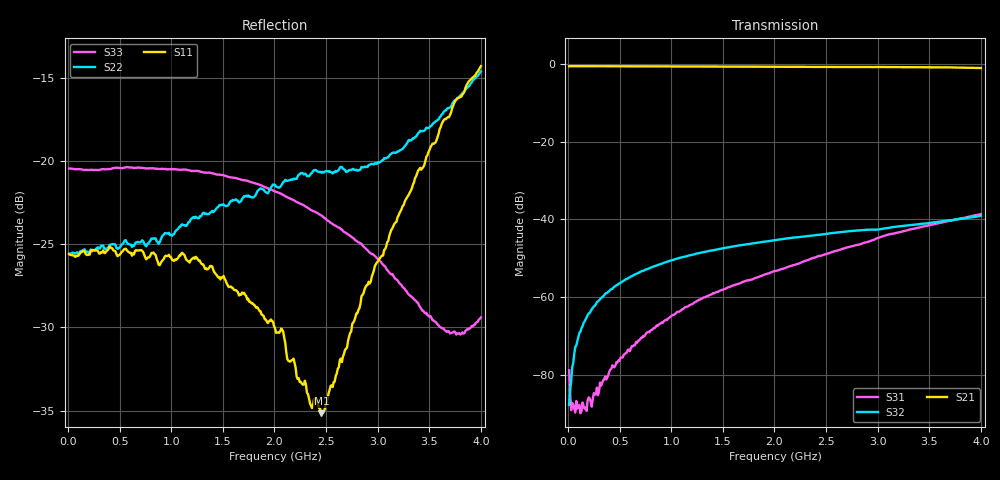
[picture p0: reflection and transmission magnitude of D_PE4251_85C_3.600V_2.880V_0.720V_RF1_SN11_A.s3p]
! Device ID: PE4251_SoldCshunt_081809
! Dir: c:\Test Bench Repositories\Bench_Software_CVI_Version_8\trunk\PSC 4Port_VNA Bench\datalog\4250\TEST\PE4251_SoldCshunt_081809\85C\3p600000\RF1
! Serial: 11
! Insertion: A
! Temp: 85C
! VDD: 3.600
! Control_Hi: 80.000
! Control_Lo: 20.000
! Logic State: RF1
! Port 1: RFC
! Port 2: RF1
! Port 3: RF2
! V1 = 0.72
! V2 = 2.88
! V3 = 0.72
! IDD: 5.518780e-05
! FILE NAME
! DATE 08/18/09  20:17
! CORRECTED  DATA
#  Hz  S  RI  R  50.00
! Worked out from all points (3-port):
!   401 points, 10 MHz to 4 GHz, reference 50 ohm
!   strongest paths, dB at 10 MHz, 1.008 GHz, 2.005 GHz, 3.002 GHz, 4 GHz:
!     S21: -0.6, -0.7, -0.8, -0.8, -1.1
!     S32: -87.7, -50.5, -45.4, -42.6, -39.1
!     S31: -78.8, -64.7, -53.3, -44.8, -38.6
!   lowest |S11| = -35.2 dB at 2.454 GHz (marker M1), VSWR 1.04, Z = 49.9 - j1.74 ohm
!   |S11| at or under -10 dB: start of sweep to end of sweep
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1e7  0.0526 0.000196  0.9309 -0.0035  8e-05 -2.85e-05
     0.9305 -0.00483  0.0525 0.000111  8.77e-05 -4.46e-05
     0.00011 3.15e-05  3.14e-05 -2.66e-05  0.0951 -0.000197
8.98e7  0.0521 -0.00168  0.9321 -0.0316  2.79e-05 -2.07e-05
        0.9314 -0.0315  0.0532 -0.00147  5.13e-05 0.000271
        2.69e-05 -2.53e-05  3.39e-05 0.000271  0.0947 -0.00193
1.696e8  0.0527 -0.000111  0.9298 -0.0584  1.66e-05 -3.75e-05
         0.9296 -0.0578  0.0537 3.84e-05  5.3e-05 0.000517
         1.05e-05 -3.66e-05  6.16e-05 0.000513  0.0942 -0.00379
3.79075e8  0.0537 -0.00419  0.9216 -0.127  -5.72e-05 -6.99e-05
           0.9208 -0.1271  0.0542 -0.00332  0.000103 0.00113
           -5.84e-05 -7.12e-05  9.56e-05 0.00113  0.0941 -0.00983
4.78825e8  0.0515 -0.00605  0.9148 -0.1604  -0.00012 -7.59e-05
           0.9144 -0.1608  0.0542 -0.00586  0.000146 0.00144
           -0.000116 -8.71e-05  0.000139 0.00143  0.0949 -0.012
1.14715e9  0.0472 -0.0178  0.8482 -0.3678  -0.000737 -7.79e-05
           0.848 -0.3673  0.0608 -0.0197  0.000556 0.00332
           -0.000745 -7.49e-05  0.000559 0.00332  0.0911 -0.0241
2.005e9  0.0259 -0.0179  0.7026 -0.5829  -0.00215 0.000146
         0.7029 -0.5828  0.0717 -0.0456  0.000988 0.0053
         -0.00215 0.000154  0.000986 0.0053  0.0751 -0.0308
2.453875e9  -0.000309 -0.0174  0.6104 -0.6739  -0.00341 0.000249
            0.6092 -0.6744  0.0618 -0.0687  0.00104 0.00628
            -0.00341 0.000239  0.00104 0.0063  0.0608 -0.0321
3.650875e9  -0.1122 -0.0734  0.2832 -0.8554  -0.00886 0.00278
            0.2848 -0.854  -0.0617 -0.1279  -0.000114 0.00954
            -0.00888 0.00275  -0.000114 0.00957  0.00533 -0.0305
4e9  -0.1762 -0.0793  0.1579 -0.8729  -0.0108 0.00441
     0.1571 -0.8697  -0.1367 -0.1268  -0.000728 0.011
     -0.0109 0.00434  -0.000772 0.0111  -0.0156 -0.0301
